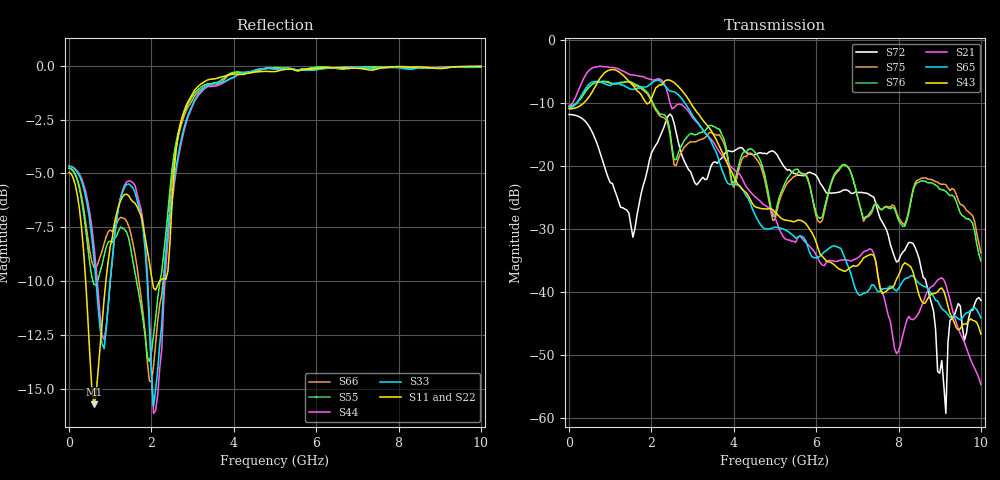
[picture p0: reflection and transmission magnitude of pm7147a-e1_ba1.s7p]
# GHz S DB R 50
! S-Parameters data
! Freq  dbS11  angS11  dbS12  angS12  dbS13  angS13  dbS14  angS14
!  dbS15  angS15  dbS16  angS16  dbS17  angS17  dbS21  angS21
!  dbS22  angS22  dbS23  angS23  dbS24  angS24  dbS25  angS25
!  dbS26  angS26  dbS27  angS27  dbS31  angS31  dbS32  angS32
!  dbS33  angS33  dbS34  angS34  dbS35  angS35  dbS36  angS36
!  dbS37  angS37  dbS41  angS41  dbS42  angS42  dbS43  angS43
!  dbS44  angS44  dbS45  angS45  dbS46  angS46  dbS47  angS47
!  dbS51  angS51  dbS52  angS52  dbS53  angS53  dbS54  angS54
!  dbS55  angS55  dbS56  angS56  dbS57  angS57  dbS61  angS61
!  dbS62  angS62  dbS63  angS63  dbS64  angS64  dbS65  angS65
!  dbS66  angS66  dbS67  angS67  dbS71  angS71  dbS72  angS72
!  dbS73  angS73  dbS74  angS74  dbS75  angS75  dbS76  angS76
!  dbS77  angS77
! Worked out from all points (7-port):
!   279 points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, 1 Hz to 10 GHz, reference 50 ohm
!   strongest paths, dB at 1 Hz, 7.943 MHz, 3.05 GHz, 6.55 GHz, 10 GHz:
!     S43: -11.0, -11.0, -11.0, -36.3, -46.6
!     S65: -10.8, -10.8, -12.5, -32.9, -44.1
!     S21: -10.4, -10.4, -12.8, -35.0, -54.6
!     S76: -10.6, -10.6, -15.1, -20.5, -35.1
!     S75: -10.6, -10.6, -16.2, -20.7, -33.8
!     S72: -11.9, -11.9, -22.7, -24.2, -41.3
!   lowest |S11| = -15.7 dB at 600 MHz (marker M1), VSWR 1.39, Z = 36 + j1.34 ohm
!   |S11| at or under -10 dB: 401.9 MHz to 893.4 MHz (491.5 MHz wide, 75.9 % of centre); 2.021 GHz to 2.199 GHz (177.7 MHz wide, 8.42 % of centre)
